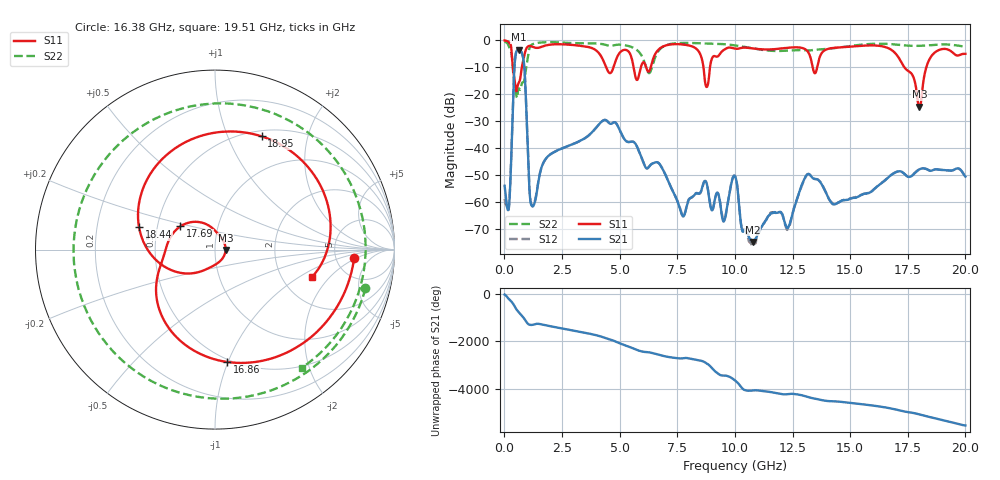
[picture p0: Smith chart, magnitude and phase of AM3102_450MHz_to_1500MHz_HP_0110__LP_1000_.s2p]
!Agilent Technologies,E8364B,MY43040894,A.07.50.67
!Agilent E8364B: A.07.50.67
!Date: Thursday, January 11, 2018 05:47:51
!Correction: S11(Full 2 Port(1,2))
!S21(Full 2 Port(1,2))
!S12(Full 2 Port(1,2))
!S22(Full 2 Port(1,2))
!S2P File: Measurements: S11, S21, S12, S22:
# Hz S  dB  R 50
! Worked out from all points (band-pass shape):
!   1601 points, 10 MHz to 20 GHz, reference 50 ohm
!   highest |S21| = -3.46 dB at 622.2 MHz (marker M1); lowest = -74.8 dB at 10.78 GHz (marker M2)
!   |S21| within 3 dB of the highest: 470.5 MHz to 811.4 MHz (340.9 MHz wide, 53.2 % of centre)
!   lowest |S11| = -24.6 dB at 18 GHz (marker M3), VSWR 1.13, Z = 56.3 - j0.166 ohm
!   |S11| at or under -10 dB: 369.3 MHz to 757.6 MHz (388.2 MHz wide, 68.9 % of centre); 4.415 GHz to 4.733 GHz (318 MHz wide, 6.95 % of centre); 17.35 GHz to 18.3 GHz (951.6 MHz wide, 5.34 % of centre)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
!   |S22| runs from -21.3 to -0.5 dB; largest |S21 - S12| = 0.0014
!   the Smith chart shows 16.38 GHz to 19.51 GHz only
!   S11 on the Smith chart (normalised r, x): 16.38 GHz: 7.49, -1.83; 16.86 GHz: 0.48, -0.99; 17.69 GHz: 0.66, +0.18; 18.44 GHz: 0.39, +0.12; 18.95 GHz: 0.56, +1.33; 19.51 GHz: 2.90, -1.31
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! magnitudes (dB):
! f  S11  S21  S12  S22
! 10 MHz  -0.1  -53.9  -58.8  -0.5
! 197.4 MHz  -0.7  -61.9  -61.8  -2.3
! 447.3 MHz  -15.1  -8.7  -8.7  -15.7
! 622.2 MHz  -15.8  -3.5  -3.5  -17.8
! 847.1 MHz  -6.3  -8.5  -8.5  -15.4
! 1.209 GHz  -2.4  -61.5  -61.1  -1.5
! 3.346 GHz  -2.1  -37.0  -37.0  -1.1
! 6.682 GHz  -3.5  -45.4  -45.4  -4.0
! 7.744 GHz  -1.6  -65.2  -65.1  -1.0
! 8.781 GHz  -17.3  -53.2  -53.3  -1.2
! 10.01 GHz  -3.1  -50.4  -50.3  -1.9
! 10.78 GHz  -3.0  -74.8  -76.2  -3.0
! 13.34 GHz  -8.6  -50.8  -50.7  -3.7
! 16.38 GHz  -2.2  -52.8  -52.8  -1.3
! 16.68 GHz  -3.0  -50.6  -50.7  -1.4
! 16.86 GHz  -4.0  -49.4  -49.4  -1.5
! 17.69 GHz  -12.7  -50.2  -50.1  -2.1
! 18 GHz  -24.6  -47.8  -47.8  -2.1
! 18.44 GHz  -7.1  -48.3  -48.2  -1.8
! 18.95 GHz  -3.3  -48.0  -48.1  -1.5
! 19.51 GHz  -5.0  -48.0  -48.0  -1.8
! 20 GHz  -5.0  -50.5  -50.3  -2.3
